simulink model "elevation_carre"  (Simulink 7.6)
settings: Solver=ode15s  StartTime=0.0  StopTime=0.02  RelTol=1e-3
StopFcn:
  | load sinus_carre.mat
  | plot(x(1,:),x(2,:), x(1,:),x(3,:))
  | grid
  | title('Carré d''un signal sinusoïdal')
  | xlabel('temps')
libraries: fl_lib x6, nesl_utility x6, elec_lib x2

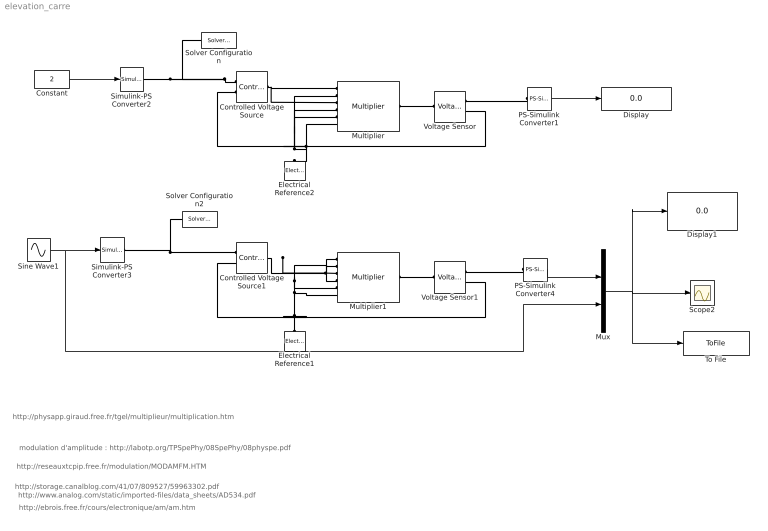
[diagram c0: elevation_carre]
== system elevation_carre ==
  note: http://www.analog.com/static/imported-files/data_sheets/AD534.pdf
  note: http://physapp.giraud.free.fr/tgel/multiplieur/multiplication.htm
  note: modulation d'amplitude : http://labotp.org/TPSpePhy/08SpePhy/08physpe.pdf
  note: http://reseauxtcpip.free.fr/modulation/MODAMFM.HTM
  note: http://storage.canalblog.com/41/07/809527/59963302.pdf
  note: http://ebrois.free.fr/cours/electronique/am/am.htm
  Constant : Constant  Value=2
  Controlled Voltage Source : fl_lib/Electrical/Electrical Sources/Controlled Voltage Source  DialogController=NetworkEngine.DynNeDlgSource  SystemSampleTime=-1  i_Log=off  v_Log=off  LocalVarNames=|i|v  LocalVarDescs=|i|v  LocalVarLogging=[0 0]
  Controlled Voltage Source1 : fl_lib/Electrical/Electrical Sources/Controlled Voltage Source  DialogController=NetworkEngine.DynNeDlgSource  SystemSampleTime=-1  i_Log=off  v_Log=off  LocalVarNames=|i|v  LocalVarDescs=|i|v  LocalVarLogging=[0 0]
  Display : Display
  Display1 : Display
  Electrical Reference1 : fl_lib/Electrical/Electrical Elements/Electrical Reference  DialogController=NetworkEngine.DynNeDlgSource  SystemSampleTime=-1  i_Log=off  LocalVarNames=|i  LocalVarDescs=|i  LocalVarLogging=[]
  Electrical Reference2 : fl_lib/Electrical/Electrical Elements/Electrical Reference  DialogController=NetworkEngine.DynNeDlgSource  SystemSampleTime=-1  i_Log=off  LocalVarNames=|i  LocalVarDescs=|i  LocalVarLogging=[]
  Multiplier : elec_lib/Integrated Circuits/Multiplier  DialogController=NetworkEngine.DynNeDlgSource  SystemSampleTime=-1  K=10 V  A=10  Rin=1e+7 Ohm  Vdiff=10 V  Rout=0.1 Ohm  Vmin=-11 V  Vmax=11 V  Vdotmax=20 V/us  f=1 MHz  V0=0 V  LocalVarLogging=[]
  Multiplier1 : elec_lib/Integrated Circuits/Multiplier  DialogController=NetworkEngine.DynNeDlgSource  SystemSampleTime=-1  K=10 V  A=10  Rin=1e+7 Ohm  Vdiff=10 V  Rout=0.1 Ohm  Vmin=-11 V  Vmax=11 V  Vdotmax=20 V/us  f=1 MHz  V0=0 V  LocalVarLogging=[]
  Mux : Mux  Inputs=2
  PS-Simulink Converter1 : nesl_utility/PS-Simulink Converter  DialogController=NetworkEngine.DynNeUtilDlgSource  SystemSampleTime=-1  PhysicalDomain=network_engine_domain  LeftPortType=input  RightPortType=output  SubClassName=ps_output  Unit=1  AffineConversion=off
  PS-Simulink Converter4 : nesl_utility/PS-Simulink Converter  DialogController=NetworkEngine.DynNeUtilDlgSource  SystemSampleTime=-1  PhysicalDomain=network_engine_domain  LeftPortType=input  RightPortType=output  SubClassName=ps_output  Unit=1  AffineConversion=off
  Scope2 : Scope
  Simulink-PS Converter2 : nesl_utility/Simulink-PS Converter  DialogController=NetworkEngine.DynNeUtilDlgSource  SystemSampleTime=-1  PhysicalDomain=network_engine_domain  LeftPortType=input  RightPortType=output  SubClassName=ps_input  Unit=1  AffineConversion=off  InputFilterTimeConstant=.001  UdotUserProvided=0
  Simulink-PS Converter3 : nesl_utility/Simulink-PS Converter  DialogController=NetworkEngine.DynNeUtilDlgSource  SystemSampleTime=-1  PhysicalDomain=network_engine_domain  LeftPortType=input  RightPortType=output  SubClassName=ps_input  Unit=1  AffineConversion=off  InputFilterTimeConstant=.001  UdotUserProvided=0
  Sine Wave1 : Sin  Frequency=2*pi*60  SampleTime=0
  Solver Configuration : nesl_utility/Solver Configuration  DialogController=NetworkEngine.DynNeUtilDlgSource  SystemSampleTime=-1  PhysicalDomain=network_engine_domain  LeftPortType=input  RightPortType=generic  SubClassName=solver  Accelerate=off  Profile=off  ResidualTolerance=1e-9  MaxNonlinIter=12  MaxModeIter=2  DoFixedCost=off  UseLocalSampling=off  DoDC=off  LinearAlgebra=Sparse  LocalSolverSampleTime=.001  LocalSolverChoice=NE_BACKWARD_EULER_ADVANCER  UseLocalSolver=off
  Solver Configuration2 : nesl_utility/Solver Configuration  DialogController=NetworkEngine.DynNeUtilDlgSource  SystemSampleTime=-1  PhysicalDomain=network_engine_domain  LeftPortType=input  RightPortType=generic  SubClassName=solver  Accelerate=off  Profile=off  ResidualTolerance=1e-9  MaxNonlinIter=12  MaxModeIter=2  DoFixedCost=off  UseLocalSampling=off  DoDC=off  LinearAlgebra=Sparse  LocalSolverSampleTime=.001  LocalSolverChoice=NE_BACKWARD_EULER_ADVANCER  UseLocalSolver=off
  To File : ToFile  Filename=sinus_carre  MatrixName=x
  Voltage Sensor : fl_lib/Electrical/Electrical Sensors/Voltage Sensor  DialogController=NetworkEngine.DynNeDlgSource  SystemSampleTime=-1  i1_Log=off  v1_Log=off  LocalVarNames=|i1|v1  LocalVarDescs=|i1|v1  LocalVarLogging=[0 0]
  Voltage Sensor1 : fl_lib/Electrical/Electrical Sensors/Voltage Sensor  DialogController=NetworkEngine.DynNeDlgSource  SystemSampleTime=-1  i1_Log=off  v1_Log=off  LocalVarNames=|i1|v1  LocalVarDescs=|i1|v1  LocalVarLogging=[0 0]
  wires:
  PS-Simulink Converter1/1 -> Display/1
  Constant/1 -> Simulink-PS Converter2/1
  Sine Wave1/1 -> Simulink-PS Converter3/1, Mux/2
  PS-Simulink Converter4/1 -> Mux/1
  Mux/1 -> Scope2/1, Display1/1, To File/1
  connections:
  Controlled Voltage Source/RConn1 -- Simulink-PS Converter2/RConn1 -- Solver Configuration/RConn1
  Controlled Voltage Source/LConn1 -- Multiplier/LConn3 -- Multiplier/LConn1
  Controlled Voltage Source/RConn2 -- Voltage Sensor/RConn2 -- Electrical Reference2/LConn1 -- Multiplier/LConn2 -- Multiplier/LConn4 -- Multiplier/LConn5 -- Multiplier/LConn6
  Multiplier/RConn1 -- Voltage Sensor/LConn1
  PS-Simulink Converter1/LConn1 -- Voltage Sensor/RConn1
  Multiplier1/LConn3 -- Controlled Voltage Source1/LConn1 -- Multiplier1/LConn1
  Multiplier1/LConn2 -- Controlled Voltage Source1/RConn2 -- Electrical Reference1/LConn1 -- Voltage Sensor1/RConn2 -- Multiplier1/LConn6 -- Multiplier1/LConn5 -- Multiplier1/LConn4
  PS-Simulink Converter4/LConn1 -- Voltage Sensor1/RConn1
  Multiplier1/RConn1 -- Voltage Sensor1/LConn1
  Controlled Voltage Source1/RConn1 -- Simulink-PS Converter3/RConn1 -- Solver Configuration2/RConn1
